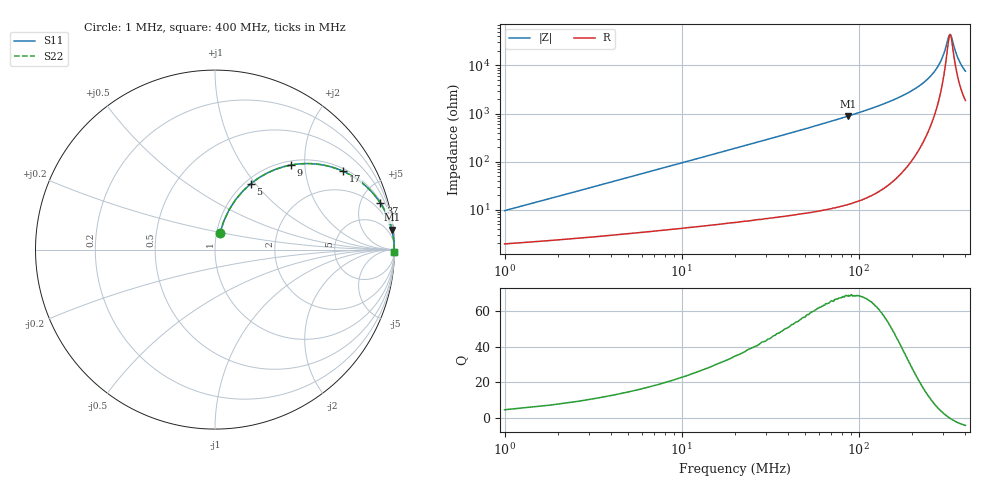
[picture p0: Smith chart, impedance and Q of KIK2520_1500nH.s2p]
!version-2
!date-01.2022
!Series
# MHz S RI R 50
!Freq ReS11 ImS11 ReS21 ImS21 ReS12 ImS12 ReS22 ImS22
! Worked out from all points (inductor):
!   500 points, 1 MHz to 400 MHz, reference 50 ohm
!   read as one part in series: L = 1.5 uH near 2.6 MHz
!   highest Q = 68.4 at 87.4 MHz (marker M1), where L = 1.61 uH
!   self-resonance near 327.5 MHz
!   S11 on the Smith chart (normalised r, x): 1 MHz: 1.04, +0.19; 5 MHz: 1.06, +0.94; 9 MHz: 1.08, +1.70; 17 MHz: 1.10, +3.21; 37 MHz: 1.15, +7.06; 400 MHz: open
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1  0.0275 0.0899  0.9725 -0.0899  0.9725 -0.0899  0.0275 0.0899
3.4  0.1134 0.2764  0.8866 -0.2764  0.8866 -0.2764  0.1134 0.2764
5  0.1982 0.3662  0.8018 -0.3662  0.8018 -0.3662  0.1982 0.3662
9  0.4229 0.4712  0.5771 -0.4712  0.5771 -0.4712  0.4229 0.4712
13  0.5977 0.4721  0.4023 -0.4721  0.4023 -0.4721  0.5977 0.4721
17  0.7148 0.4359  0.2852 -0.4359  0.2852 -0.4359  0.7148 0.4359
25  0.8427 0.3516  0.1573 -0.3516  0.1573 -0.3516  0.8427 0.3516
37  0.9213 0.2592  0.0787 -0.2592  0.0787 -0.2592  0.9213 0.2592
68.2  0.9762 0.1449  0.0238 -0.1449  0.0238 -0.1449  0.9762 0.1449
87.4  0.9859 0.111  0.0141 -0.111  0.0141 -0.111  0.9859 0.111
134  0.9946 0.0656  0.00545 -0.0656  0.00545 -0.0656  0.9946 0.0656
201  0.9977 0.0328  0.00227 -0.0328  0.00227 -0.0328  0.9977 0.0328
239  0.9981 0.0209  0.00186 -0.0209  0.00186 -0.0209  0.9981 0.0209
267  0.9982 0.0135  0.00183 -0.0135  0.00183 -0.0135  0.9982 0.0135
299  0.998 0.00607  0.00199 -0.00607  0.00199 -0.00607  0.998 0.00607
324  0.9978 0.000781  0.00224 -0.000781  0.00224 -0.000781  0.9978 0.000781
329  0.9977 -0.000161  0.00229 0.000161  0.00229 0.000161  0.9977 -0.000161
334  0.9976 -0.00109  0.00235 0.00109  0.00235 0.00109  0.9976 -0.00109
348  0.9975 -0.0038  0.00254 0.0038  0.00254 0.0038  0.9975 -0.0038
360  0.9973 -0.00597  0.00272 0.00597  0.00272 0.00597  0.9973 -0.00597
380  0.997 -0.00944  0.00305 0.00944  0.00305 0.00944  0.997 -0.00944
400  0.9966 -0.0127  0.00341 0.0127  0.00341 0.0127  0.9966 -0.0127
